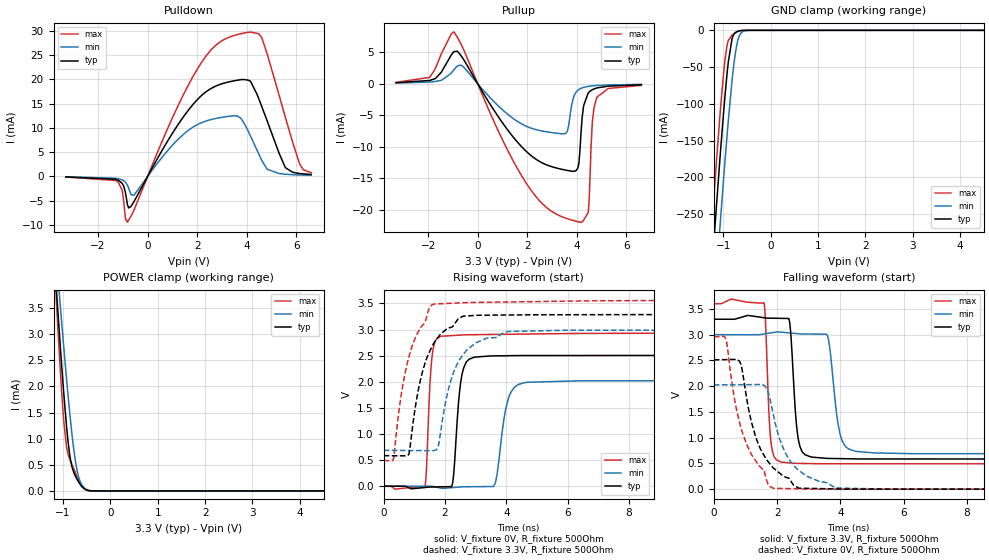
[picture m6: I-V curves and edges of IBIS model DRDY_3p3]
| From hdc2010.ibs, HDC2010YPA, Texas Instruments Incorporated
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[Model]   DRDY_3p3
Model_type   I/O
Polarity   Non-Inverting
Enable   Active-Low
Vinl = 0.99
Vinh = 2.31
Vmeas = 1.65
Vref = 3.3
Cref = 15pF
Rref = 500
|   typ   min   max
|   (nom PVT)   (slow PVT)   (fast PVT)
C_comp   0.808p   0.802p   0.818p
|C_comp (High state)   0.850p   0.838p   0.867p
|C_comp (Low state)   0.808p   0.802p   0.818p
[Model spec]
|subparameter
Vinl   0.99   0.90   1.08
Vinh   2.31   2.10   2.52
[Voltage Range]   3.3   3   3.6
[Temperature Range]   27   125   -40
[Pullup Reference]   3.3   3   3.6
[Pulldown Reference]   0   0   -0
[Power Clamp Reference]   3.3   3   3.6
[GND Clamp Reference]   0   0   0
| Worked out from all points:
|   slope of the pulldown table from 0 to 0.495 V, typ, clamps not added: 108 ohm
|   slope of the pullup table from 0 to 0.495 V, typ, clamps not added: 154 ohm
|   GND clamp passes 1 mA (typ) near -0.68 V on its own axis
|   POWER clamp passes 1 mA (typ) near -0.90 V on its own axis
|   falling waveform, V_fixture 3.3V, R_fixture 500Ohm: 20-80 % time 174ps typ, 261ps min, 125ps max; typ from 3.3 V to 0.585 V
|   rising waveform, V_fixture 0V, R_fixture 500Ohm: 20-80 % time 199ps typ, 302ps min, 143ps max; typ from 0 V to 2.51 V
|   rising waveform, V_fixture 3.3V, R_fixture 500Ohm: 20-80 % time 716ps typ, 722ps min, 706ps max; typ from 0.585 V to 3.3 V
|   falling waveform, V_fixture 0V, R_fixture 500Ohm: 20-80 % time 784ps typ, 791ps min, 772ps max; typ from 2.51 V to 0 V
[Pulldown]
|   Voltage   I(typ)   I(min)   I(max)
-3.3V     -95.85uA   -72.7uA    -114.7uA
-1.221V   -692.9uA   -422.5uA   -1.043mA
-1.033V   -1.374mA   -686.3uA   -2.782mA
-815.1mV  -5.756mA   -1.774mA   -9.426mA
-567.6mV  -5.34mA    -3.901mA   -7.129mA
2.135V    16.49mA    11mA       23.19mA
3.62V     19.84mA    12.46mA    29.24mA
4.145V    19.62mA    8.401mA    29.75mA
4.61V     14.35mA    3.246mA    28.53mA
5.551V    1.885mA    463uA      12.29mA
6.135V    597.8uA    304.6uA    2.57mA
6.6V      407.9uA    239.9uA    770.1uA
[GND Clamp]
|   Voltage   I(typ)   I(min)   I(max)
-3.3V     -2.325A    -2.409A    -2.272A
-1.241V   -326.2mA   -420.2mA   -265.5mA
-1.211V   -299.2mA   -393.2mA   -238.5mA
-1.132V   -228.4mA   -322.1mA   -168.2mA
-1.073V   -176.9mA   -269.9mA   -118.1mA
-983.4mV  -104.4mA   -194.3mA   -52.07mA
-924mV    -61.84mA   -146.5mA   -22.26mA
-815.1mV  -11.58mA   -68.87mA   -6.408mA
-706.2mV  -1.687mA   -17.6mA    -2.098mA
-617.1mV  -303.9uA   -3.164mA   -304.7uA
-458.7mV  -4.713uA   -93.46uA   -1.253uA
6.6V      0A         0A         0A
[Pullup]
|   Voltage   I(typ)   I(min)   I(max)
-3.3V     170.5uA    115.4uA    229.3uA
-1.934V   532.1uA    281.2uA    1.043mA
-953.7mV  5.107mA    2.26mA     8.198mA
2.373V    -12.03mA   -7.292mA   -18mA
3.571V    -13.71mA   -7.792mA   -21.34mA
4.036V    -13.38mA   -1.039mA   -21.86mA
4.155V    -8.526mA   -739.8uA   -21.95mA
4.274V    -3.439mA   -567.5uA   -21.61mA
4.452V    -1.502mA   -416.1uA   -20.44mA
4.62V     -942.7uA   -330.1uA   -6.278mA
4.798V    -667.8uA   -269.7uA   -2.213mA
6.6V      -160.5uA   -90.46uA   -246.2uA
[POWER Clamp]
|   Voltage   I(typ)   I(min)   I(max)
-3.3V     36.06mA    31.05mA    44.88mA
-1.231V   5.118mA    5.523mA    5.227mA
-1.132V   3.757mA    4.384mA    3.512mA
-1.082V   3.099mA    3.827mA    2.704mA
-1.063V   2.842mA    3.606mA    2.396mA
-983.4mV  1.865mA    2.746mA    1.327mA
-924mV    1.223mA    2.131mA    835.1uA
-854.7mV  665.7uA    1.465mA    597.8uA
-765.6mV  342.6uA    746.3uA    412uA
-696.3mV  211.9uA    364.3uA    259uA
-498.3mV  15.5uA     27.7uA     12.83uA
6.6V      0A         0A         0A
[Ramp]
R_load = 500
|   typ   min   max
dV/dt_r   1.50552/1.98484e-10   1.21346/2.9748e-10   1.77076/1.41963e-10
dV/dt_f   1.6288/1.73217e-10   1.38776/2.58041e-10   1.86461/1.25138e-10
[Falling Waveform]
V_fixture = 3.3V
V_fixture_min = 3V
V_fixture_max = 3.6V
R_fixture = 500Ohm
C_fixture = 0F
|   Time   V(typ)   V(min)   V(max)
0s        3.3V       3V         3.6V
1.583ns   3.33V      3.014V     3.621V
1.801ns   3.321V     3.035V     950.9mV
2.101ns   3.317V     3.05V      532.2mV
2.38ns    3.295V     3.035V     510.4mV
3.05ns    629.6mV    3.013V     496.5mV
3.586ns   597.6mV    2.989V     493mV
3.983ns   593.2mV    1.086V     493mV
4.445ns   588.4mV    741.1mV    493mV
19ns      585.3mV    687.1mV    492.3mV
[Rising Waveform]
V_fixture = 0V
V_fixture_min = 0V
V_fixture_max = 0V
R_fixture = 500Ohm
C_fixture = 0F
|   Time   V(typ)   V(min)   V(max)
0s        2.696nV    29.48nV    -2.287uV
1.341ns   -24.49mV   368.2uV    -10.27mV
1.572ns   -15.46mV   431.7uV    2.448V
1.856ns   -11.97mV   -35.96mV   2.868V
2.228ns   10.86mV    -27.29mV   2.884V
2.539ns   2.089V     -13.42mV   2.895V
2.945ns   2.469V     -9.124mV   2.902V
3.633ns   2.496V     49.39mV    2.907V
4.608ns   2.502V     1.984V     2.914V
19ns      2.509V     2.022V     2.951V
[Rising Waveform]
V_fixture = 3.3V
V_fixture_min = 3V
V_fixture_max = 3.6V
R_fixture = 500Ohm
C_fixture = 0F
|   Time   V(typ)   V(min)   V(max)
0s        585.2mV    687mV      492.2mV
317.5ps   583.5mV    685.8mV    515.2mV
558.3ps   582.2mV    684.9mV    1.694V
815ps     606.8mV    683.9mV    2.463V
1.193ns   2.019V     682.5mV    3.023V
1.63ns    2.733V     681.3mV    3.487V
1.771ns   2.848V     748.2mV    3.492V
2.496ns   3.226V     2.446V     3.511V
4.041ns   3.279V     2.96V      3.528V
19ns      3.296V     2.992V     3.584V
[Falling Waveform]
|Gnd
V_fixture = 0V
V_fixture_min = 0V
V_fixture_max = 0V
R_fixture = 500Ohm
C_fixture = 0F
|   Time   V(typ)   V(min)   V(max)
0s        2.511V     2.025V     2.96V
387.7ps   2.516V     2.027V     2.9V
818.8ps   2.478V     2.029V     1.284V
1.313ns   1.037V     2.031V     561mV
1.685ns   559.5mV    1.942V     146.3mV
1.872ns   416.5mV    1.478V     20.11mV
2.097ns   303.2mV    946.4mV    14.7mV
2.445ns   147mV      519mV      9.852mV
3.935ns   3.653mV    20.9mV     635.3uV
19ns      92.82uV    67.15uV    78.32uV
